| IBIS file k66_180_144lqfp_derated.ibs generated by Viper version: 2014.12.11
[IBIS Ver]   4.2
[Comment Char]   |_char
[File Name]   k66_180_144lqfp_derated.ibs
[File Rev]   1.0
[Date]   Thu Dec 17 11:43:14 2015
[Source]   FSL Viper 2014.12.11
[Notes]
[Disclaimer] IMPORTANT NOTICE
  This information is provided on an AS IS basis and without warranty.
  IN NO EVENT SHALL Freescale BE LIABLE FOR INCIDENTAL OR CONSEQUENTIAL
  DAMAGES ARISING FROM USE OF THIS INFORMATION. THIS DISCLAIMER OF
  WARRANTY EXTENDS TO THE USER OF THE INFORMATION, AND TO THEIR CUSTOMERS
  OR USERS OF PRODUCTS  AND IS IN LIEU OF ALL WARRANTIES WHETHER EXPRESS,
  IMPLIED, OR STATUTORY, INCLUDING IMPLIED WARRANTIES OF MERCHANTABILITY
  OR FITNESS FOR PARTICULAR PURPOSE.
  Freescale does not represent or warrant that the information furnished
  hereunder is free of infringement of any third party patents,
  copyrights, trade secrets, or other intellectual property rights.
  Freescale does not represent or warrant that the information is free of
  defect, or that it meets any particular standard, requirements or need
  of the user of the infomation or their customers.
  Freescale reserves the right to change the information in this file
  without notice.
   http://www.freescale.com
[Copyright]   (C) Copyright Freescale 2004 - 2015, All Rights Reserved.
|   k66_144lqfp
[Component]   k66_144lqfp
[Manufacturer]   FREESCALE
[Package]
| variable   typ   min   max
R_pkg   0.19858   0.13084   0.24148
L_pkg   6.875e-9   4.9e-9   8.329e-9
C_pkg   1.219e-12   8.712e-13   1.463e-12
[Pin] signal_name   model_name   R_pin   L_pin   C_pin
1   PTE0   p_io_fast_84u3v_6m   0.21841   7.994e-9  1.086e-12
2   PTE1   p_io_fast_84u3v_6m   0.21026   7.594e-9  1.405e-12
3   PTE2   p_io_fast_84u3v_6m   0.20847   7.418e-9  1.405e-12
4   PTE3   p_io_fast_84u3v_6m   0.20973   7.107e-9  1.348e-12
5   VDD_0   POWER   0.15175   5.891e-9  1.346e-12
6   VSS_0   GND   NA   NA   NA
7   PTE4   p_io_fast_84u3v_6m   0.21096   6.184e-9  1.181e-12
8   PTE5   p_io_fast_84u3v_6m   0.20069   6.659e-9  1.25e-12
9   PTE6   p_io_fast_84u3v_6m   0.19693   6.721e-9  1.218e-12
10   PTE7   p_io_fast_84u3v_6m   0.19456   6.711e-9  1.171e-12
11   PTE8   p_io_fast_84u3v_6m   0.19383   6.699e-9  1.126e-12
12   PTE9   p_io_fast_84u3v_6m   0.19212   6.489e-9  1.038e-12
13   PTE10   p_io_fast_84u3v_6m   0.19207   6.373e-9  1.136e-12
14   PTE11   p_io_fast_84u3v_6m   0.19367   6.261e-9  1.138e-12
15   PTE12   p_io_fast_84u3v_6m   0.19709   6.039e-9  1.1e-12
16   VDD_1   POWER   0.13849   4.9e-9   1.127e-12
17   VSS_1   GND   NA   NA   NA
18   USB0VSS   GND   NA   NA   NA
19   USB0DP   NC   0.20642   5.586e-9  1.006e-12
20   USB0DM   NC   0.19901   6.029e-9  1.133e-12
21   VREGOUT   POWER   0.13139   5.644e-9  1.181e-12
22   VREGIN0   POWER   0.13084   5.802e-9  1.128e-12
23   VREGIN1   POWER   0.13087   5.905e-9  1.219e-12
24   USB1VSS   GND   0.13091   6.012e-9  1.177e-12
25   USB1DP   NC   0.19605   6.706e-9  1.24e-12
26   USB1DM   NC   0.19837   6.925e-9  1.247e-12
27   USB1VBUS   POWER   0.13397   6.405e-9  1.22e-12
28   ADC0DM0_ADC1DM3   NC   0.19436   7.041e-9  1.17e-12
29   ADC1DP0_ADC0DP3   NC   0.19505   7.129e-9  1.217e-12
30   ADC1DM0_ADC0DM3   NC   0.19627   7.248e-9  1.362e-12
31   VDDA   POWER   0.19789   7.362e-9  1.405e-12
32   VREFH   POWER   0.19979   7.453e-9  1.277e-12
33   VREFL   NC   0.20279   7.575e-9  1.322e-12
34   VSSA   GND   0.20557   7.708e-9  1.435e-12
35   ADC1SE16_CMP2IN2_ADC0SE22   NC   0.20989   7.842e-9  1.463e-12
36   ADC0SE16_CMP1IN2_ADC0SE21   NC   0.22459   8.329e-9  1.193e-12
37   VREFOUT_CMP1IN5_CMP0IN5_ADC1SE18   NC   0.22612   8.288e-9  1.132e-12
38   DAC0OUT_CMP1IN3_ADC0SE23   NC   0.22077   7.993e-9  1.431e-12
39   DAC1OUT_CMP0IN4_CMP2IN3_ADC1SE23   NC   0.21663   7.872e-9  1.413e-12
40   XTAL32   NC   0.2377   8.098e-9  1.431e-12
41   EXTAL32   NC   0.23437   7.821e-9  1.387e-12
42   VBAT   POWER   0.2332   7.389e-9  1.353e-12
43   VDD_2   POWER   0.1662   6.086e-9  1.394e-12
44   VSS_2   GND   NA   NA   NA
45   PTE24   p_io_fast_84u3v_6m   0.24148   6.355e-9  1.261e-12
46   PTE25   p_io_fast_84u3v_6m   0.22683   6.868e-9  1.265e-12
47   PTE26   p_io_fast_84u3v_6m   0.21975   7.055e-9  1.219e-12
48   PTE27   p_io_fast_84u3v_6m   0.21407   6.963e-9  1.222e-12
49   PTE28   p_io_fast_84u3v_6m   0.21097   6.913e-9  1.192e-12
50   PTA0   p_io_fast_84u3v_6m   0.20817   6.846e-9  1.161e-12
51   PTA1   p_io_fast_84u3v_6m   0.20617   6.766e-9  1.106e-12
52   PTA2   p_io_fast_84u3v_6m   0.2045   6.656e-9  1.144e-12
53   PTA3   p_io_fast_84u3v_6m   0.20359   6.569e-9  1.147e-12
54   PTA4   p_io_flt_84u3v_6m   0.20444   6.415e-9  1.117e-12
55   PTA5   p_io_fast_84u3v_6m   0.20686   6.194e-9  1.123e-12
56   VDD_3   POWER   0.14623   5.036e-9  1.164e-12
57   VSS_3   GND   NA   NA   NA
58   PTA6   p_io_fast_84u3v_6m   0.2117   5.761e-9  1.158e-12
59   PTA7   p_io_fast_84u3v_6m   0.203   6.303e-9  1.125e-12
60   PTA8   p_io_fast_84u3v_6m   0.19874   6.513e-9  1.17e-12
61   PTA9   p_io_fast_84u3v_6m   0.19739   6.647e-9  1.155e-12
62   PTA10   p_io_fast_84u3v_6m   0.19835   6.882e-9  1.266e-12
63   PTA11   p_io_fast_84u3v_6m   0.19868   6.952e-9  1.245e-12
64   PTA12   p_io_fast_84u3v_6m   0.20027   7.068e-9  1.233e-12
65   PTA13   p_io_fast_84u3v_6m   0.20197   7.15e-9   1.265e-12
66   PTA14   p_io_fast_84u3v_6m   0.2046   7.27e-9   1.377e-12
67   PTA15   p_io_fast_84u3v_6m   0.20756   7.325e-9  1.404e-12
68   PTA16   p_io_fast_84u3v_6m   0.21228   7.33e-9   1.38e-12
69   PTA17   p_io_fast_84u3v_6m   0.21966   7.225e-9  1.337e-12
70   VDD_4   POWER   0.16123   6.16e-9   1.44e-12
71   VSS_4   GND   NA   NA   NA
72   PTA18   p_io_fast_84u3v_6m   0.23986   6.914e-9  1.173e-12
73   PTA19   p_io_fast_84u3v_6m   0.22064   7.978e-9  1.128e-12
74   RESETB   p_vpp_84u3v_6m   0.21453   7.795e-9  1.412e-12
75   PTA24   p_io_fast_84u3v_6m   0.21216   7.731e-9  1.388e-12
76   PTA25   p_io_fast_84u3v_6m   0.20948   7.642e-9  1.439e-12
77   PTA26   p_io_fast_84u3v_6m   0.2069   7.599e-9  1.367e-12
78   PTA27   p_io_fast_84u3v_6m   0.20239   7.345e-9  1.258e-12
79   PTA28   p_io_fast_84u3v_6m   0.1997   7.249e-9  1.341e-12
80   PTA29   p_io_fast_84u3v_6m   0.19753   7.14e-9   1.202e-12
81   PTB0   p_io_fast_hd_84u3v_6m   0.19889   7.122e-9  1.202e-12
82   PTB1   p_io_fast_hd_84u3v_6m   0.19751   7.034e-9  1.175e-12
83   PTB2   p_io_fast_84u3v_6m   0.19706   7.002e-9  1.152e-12
84   PTB3   p_io_fast_84u3v_6m   0.19487   6.832e-9  1.173e-12
85   PTB4   p_io_fast_84u3v_6m   0.19718   6.794e-9  1.112e-12
86   PTB5   p_io_fast_84u3v_6m   0.19572   6.701e-9  1.11e-12
87   PTB6   p_io_fast_84u3v_6m   0.19463   6.611e-9  1.073e-12
88   PTB7   p_io_fast_84u3v_6m   0.19441   6.552e-9  1.059e-12
89   PTB8   p_io_fast_84u3v_6m   0.19453   6.477e-9  1.136e-12
90   PTB9   p_io_fast_84u3v_6m   0.19523   6.341e-9  1.036e-12
91   PTB10   p_io_fast_84u3v_6m   0.19696   6.213e-9  1.049e-12
92   PTB11   p_io_fast_84u3v_6m   0.20036   5.925e-9  9.911e-13
93   VSS_6   GND   NA   NA   NA
94   VDD_6   POWER   0.1391   5.138e-9  1.155e-12
95   PTB16   p_io_fast_84u3v_6m   0.19766   6.202e-9  1.106e-12
96   PTB17   p_io_fast_84u3v_6m   0.19444   6.415e-9  1.124e-12
97   PTB18   p_io_fast_84u3v_6m   0.19359   6.55e-9   1.123e-12
98   PTB19   p_io_fast_84u3v_6m   0.19456   6.748e-9  1.13e-12
99   PTB20   p_io_fast_84u3v_6m   0.1952   6.875e-9  1.299e-12
100   PTB21   p_io_fast_84u3v_6m   0.19665   6.954e-9  1.288e-12
101   PTB22   p_io_fast_84u3v_6m   0.19844   7.03e-9   1.243e-12
102   PTB23   p_io_fast_84u3v_6m   0.20125   7.145e-9  1.315e-12
103   PTC0   p_io_fast_84u3v_6m   0.20427   7.208e-9  1.375e-12
104   PTC1   p_io_fast_84u3v_6m   0.20893   7.224e-9  1.38e-12
105   PTC2   p_io_fast_84u3v_6m   0.21555   7.112e-9  1.397e-12
106   PTC3   p_io_fast_hd_84u3v_6m   0.22791   6.592e-9  1.39e-12
107   VSS_7   GND   NA   NA   NA
108   VDD_7   POWER   0.16613   6.238e-9  1.209e-12
109   PTC4   p_io_fast_hd_84u3v_6m   0.22027   7.899e-9  1.096e-12
110   PTC5   p_io_fast_84u3v_6m   0.21544   7.741e-9  1.41e-12
111   PTC6   p_io_fast_84u3v_6m   0.21032   7.598e-9  1.356e-12
112   PTC7   p_io_fast_84u3v_6m   0.20793   7.512e-9  1.368e-12
113   PTC8   p_io_fast_84u3v_6m   0.20576   7.469e-9  1.328e-12
114   PTC9   p_io_fast_84u3v_6m   0.20242   7.272e-9  1.312e-12
115   PTC10   p_io_fast_84u3v_6m   0.20005   7.132e-9  1.298e-12
116   PTC11   p_io_fast_84u3v_6m   0.19877   7.013e-9  1.226e-12
117   PTC12   p_io_fast_84u3v_6m   0.19828   6.903e-9  1.252e-12
118   PTC13   p_io_fast_84u3v_6m   0.19856   6.702e-9  1.141e-12
119   PTC14   p_io_fast_84u3v_6m   0.20121   6.554e-9  1.172e-12
120   PTC15   p_io_fast_84u3v_6m   0.20752   5.923e-9  1.113e-12
121   VSS_8   GND   NA   NA   NA
122   VDD_8   POWER   0.14072   5.178e-9  1.12e-12
123   PTC16   p_io_fast_84u3v_6m   0.20064   6.204e-9  1.013e-12
124   PTC17   p_io_fast_84u3v_6m   0.19835   6.416e-9  1.05e-12
125   PTC18   p_io_fast_84u3v_6m   0.19868   6.501e-9  1.033e-12
126   PTC19   p_io_fast_84u3v_6m   0.19954   6.563e-9  1.049e-12
127   PTD0   p_io_fast_84u3v_6m   0.19743   6.588e-9  1.019e-12
128   PTD1   p_io_fast_84u3v_6m   0.19617   6.577e-9  1.013e-12
129   PTD2   p_io_fast_84u3v_6m   0.19567   6.65e-9   1.051e-12
130   PTD3   p_io_fast_84u3v_6m   0.19553   6.706e-9  1.028e-12
131   PTD4   p_io_fast_hd_84u3v_6m   0.19538   6.751e-9  1.079e-12
132   PTD5   p_io_fast_hd_84u3v_6m   0.19544   6.811e-9  1.025e-12
133   PTD6   p_io_fast_hd_84u3v_6m   0.19551   6.882e-9  8.712e-13
134   VSS_10   GND   NA   NA   NA
135   VDD_10   POWER   0.133   6.499e-9  1.057e-12
136   PTD7   p_io_fast_hd_84u3v_6m   0.19903   7.105e-9  1.258e-12
137   PTD8   p_io_fast_84u3v_6m   0.1998   7.214e-9  1.231e-12
138   PTD9   p_io_fast_84u3v_6m   0.20162   7.329e-9  1.263e-12
139   PTD10   p_io_fast_84u3v_6m   0.20399   7.444e-9  1.309e-12
140   PTD11   p_io_fast_84u3v_6m   0.20676   7.561e-9  1.296e-12
141   PTD12   p_io_fast_84u3v_6m   0.20969   7.689e-9  1.331e-12
142   PTD13   p_io_fast_84u3v_6m   0.21234   7.826e-9  1.403e-12
143   PTD14   p_io_fast_84u3v_6m   0.21623   7.911e-9  1.4e-12
144   PTD15   p_io_fast_84u3v_6m   0.22062   8.131e-9  1.139e-12
[Pin Mapping]   pulldown_ref   pullup_ref
1   NC   NC
2   NC   NC
3   NC   NC
4   NC   NC
5   NC   VDD_0
6   VSS_0   NC
7   NC   NC
8   NC   NC
9   NC   NC
10   NC   NC
11   NC   NC
12   NC   NC
13   NC   NC
14   NC   NC
15   NC   NC
16   NC   VDD_1
17   VSS_1   NC
18   USB0VSS   NC
19   NC   NC
20   NC   NC
21   NC   VREGOUT
22   NC   VREGIN0
23   NC   VREGIN1
24   USB1VSS   NC
25   NC   NC
26   NC   NC
27   NC   USB1VBUS
28   NC   NC
29   NC   NC
30   NC   NC
31   NC   VDDA
32   NC   VREFH
33   NC   NC
34   VSSA   NC
35   NC   NC
36   NC   NC
37   NC   NC
38   NC   NC
39   NC   NC
40   NC   NC
41   NC   NC
42   NC   VBAT
43   NC   VDD_2
44   VSS_2   NC
45   NC   NC
46   NC   NC
47   NC   NC
48   NC   NC
49   NC   NC
50   NC   NC
51   NC   NC
52   NC   NC
53   NC   NC
54   NC   NC
55   NC   NC
56   NC   VDD_3
57   VSS_3   NC
58   NC   NC
59   NC   NC
60   NC   NC
61   NC   NC
62   NC   NC
63   NC   NC
64   NC   NC
65   NC   NC
66   NC   NC
67   NC   NC
68   NC   NC
69   NC   NC
70   NC   VDD_4
71   VSS_4   NC
72   NC   NC
73   NC   NC
74   NC   NC
75   NC   NC
76   NC   NC
77   NC   NC
78   NC   NC
79   NC   NC
80   NC   NC
81   NC   NC
82   NC   NC
83   NC   NC
84   NC   NC
85   NC   NC
86   NC   NC
87   NC   NC
88   NC   NC
89   NC   NC
90   NC   NC
91   NC   NC
92   NC   NC
93   VSS_6   NC
94   NC   VDD_6
95   NC   NC
96   NC   NC
97   NC   NC
98   NC   NC
99   NC   NC
100   NC   NC
101   NC   NC
102   NC   NC
103   NC   NC
104   NC   NC
105   NC   NC
106   NC   NC
107   VSS_7   NC
108   NC   VDD_7
109   NC   NC
110   NC   NC
111   NC   NC
112   NC   NC
113   NC   NC
114   NC   NC
115   NC   NC
116   NC   NC
117   NC   NC
118   NC   NC
119   NC   NC
120   NC   NC
121   VSS_8   NC
122   NC   VDD_8
123   NC   NC
124   NC   NC
125   NC   NC
126   NC   NC
127   NC   NC
128   NC   NC
129   NC   NC
130   NC   NC
131   NC   NC
132   NC   NC
133   NC   NC
134   VSS_10   NC
135   NC   VDD_10
136   NC   NC
137   NC   NC
138   NC   NC
139   NC   NC
140   NC   NC
141   NC   NC
142   NC   NC
143   NC   NC
144   NC   NC
|*   Model Selector   *
[Model Selector] p_io_fast_84u3v_6m
p_io_fast_84u3v_6m_sre0   io, without slew rate
p_io_fast_84u3v_6m_sre1   io, with slew rate
[Model Selector] p_io_fast_hd_84u3v_6m
p_io_fast_hd_84u3v_6m_obe1dse0sre0   io 5mA, without slew rate
p_io_fast_hd_84u3v_6m_obe1dse0sre1   io 5mA, with slew rate
p_io_fast_hd_84u3v_6m_obe1dse1sre0   io 20mA, without slew rate
p_io_fast_hd_84u3v_6m_obe1dse1sre1   io 20mA, with slew rate
[Model Selector] p_io_flt_84u3v_6m
p_io_flt_84u3v_6m_sre0   io_flt, without slew rate
p_io_flt_84u3v_6m_sre1   io_flt, with slew rate
| End [Component] k66_144lqfp
| Models and submodels in the file (9): p_io_fast_84u3v_6m_sre0 (I/O), p_io_fast_84u3v_6m_sre1 (I/O), p_io_fast_hd_84u3v_6m_obe1dse0sre0 (I/O), p_io_fast_hd_84u3v_6m_obe1dse0sre1 (I/O), p_io_fast_hd_84u3v_6m_obe1dse1sre0 (I/O), p_io_fast_hd_84u3v_6m_obe1dse1sre1 (I/O), p_io_flt_84u3v_6m_sre0 (I/O), p_io_flt_84u3v_6m_sre1 (I/O), p_vpp_84u3v_6m (I/O_open_drain)
